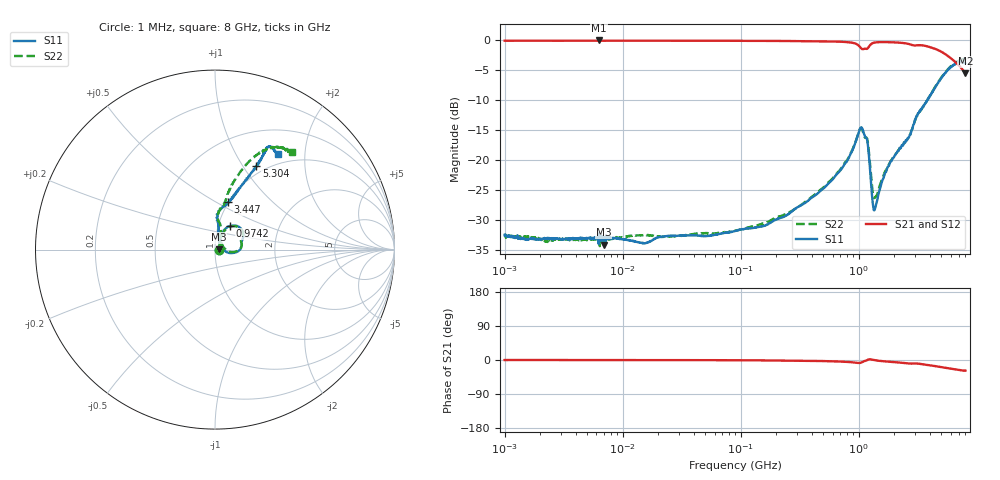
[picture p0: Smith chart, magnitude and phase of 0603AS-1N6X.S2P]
!s-Parameter Generated by FASTRON Sdn. Bhd.
!FASTRON P/N : 0603AS-1N6X
!Keysight Technologies: E5071C_MY46733604_B.14.02
!Date: Tue Oct 24 10:20:23 2023
!Version  :Rev01  Tue Oct 24 10:20:23 2023
!Data & Calibration Information:
!Freq  S11:SOLT2(ON)  S21:SOLT2(ON)  S12:SOLT2(ON)  S22:SOLT2(ON)
!PortZ  Port1:50+j0  Port2:50+j0
!When reading reference impedance value at option line is always used.
! Remarks : This data is being provided solely for informational purposes.
# Hz S dB R 50
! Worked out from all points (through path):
!   1601 points, 1 MHz to 8 GHz, reference 50 ohm
!   highest |S21| = -0.16 dB at 6.301 MHz (marker M1); lowest = -5.6 dB at 8 GHz (marker M2)
!   group delay of S21, straight-line fit = 9.86 ps
!   lowest |S11| = -34.1 dB at 6.912 MHz (marker M3), VSWR 1.04, Z = 52 + j0.239 ohm
!   |S11| at or under -10 dB: start of sweep to 3.812 GHz
!   |S22| runs from -34.4 to -3.2 dB; largest |S21 - S12| = 0.0081
!   S11 on the Smith chart (normalised r, x): 1 MHz: 1.05, -0.00; 974.2 MHz: 1.14, +0.31; 3.447 GHz: 1.00, +0.57; 5.304 GHz: 0.90, +1.15; 8 GHz: 0.85, +1.50
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1000000  -32.47 -0.8  -0.20 -0.1  -0.20 0.0  -32.57 0.2
4479405  -33.04 1.9  -0.20 -0.1  -0.20 -0.0  -33.33 2.2
6301378  -32.23 0.8  -0.16 -0.1  -0.23 -0.0  -33.38 -6.3
6911657  -34.10 6.7  -0.21 -0.0  -0.22 -0.1  -33.77 4.9
1.526847e7  -33.88 -1.8  -0.19 -0.1  -0.21 -0.2  -32.54 3.8
2.00676e7  -32.88 5.8  -0.20 -0.2  -0.21 -0.1  -32.80 8.3
8.994653e7  -31.84 23.6  -0.21 -0.7  -0.22 -0.6  -31.80 21.5
1.639593e8  -30.88 33.2  -0.23 -1.0  -0.24 -1.0  -30.47 32.9
4.006501e8  -26.26 55.9  -0.28 -2.2  -0.28 -2.2  -26.14 54.9
7.032132e8  -21.70 65.8  -0.37 -4.2  -0.37 -4.2  -21.53 63.9
9.741931e8  -16.14 57.8  -0.84 -7.6  -0.85 -7.6  -16.06 55.1
1.052804e9  -14.62 36.3  -1.51 -6.6  -1.51 -6.6  -14.73 34.1
1.14826e9  -16.32 13.9  -1.54 -2.0  -1.54 -2.0  -16.34 16.5
1.210338e9  -18.64 -7.6  -1.27 1.6  -1.27 1.5  -18.10 -3.4
1.310879e9  -27.08 5.0  -0.60 0.5  -0.60 0.4  -25.30 6.1
1.365017e9  -28.30 35.4  -0.50 -0.6  -0.51 -0.7  -26.34 26.5
1.7949e9  -21.03 78.6  -0.44 -4.4  -0.44 -4.5  -20.82 71.0
2.648292e9  -16.37 83.8  -0.74 -9.2  -0.75 -9.2  -16.26 81.2
3.446699e9  -11.28 74.5  -0.97 -11.1  -0.98 -11.1  -11.40 78.1
5.304358e9  -5.70 63.6  -2.33 -20.2  -2.32 -20.3  -5.62 68.9
6.881909e9  -3.83 62.6  -4.13 -25.6  -4.12 -25.9  -3.65 60.6
8e9  -3.95 56.7  -5.64 -28.1  -5.63 -28.5  -3.17 51.8
